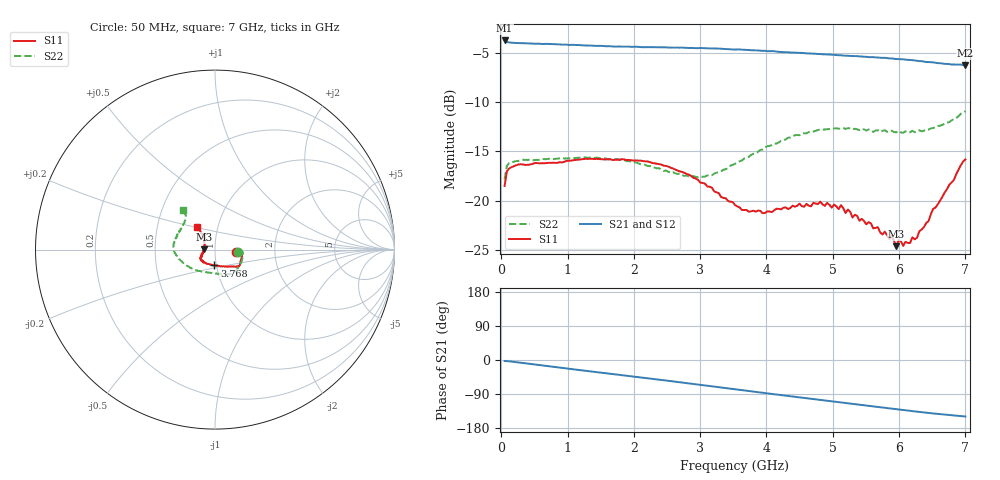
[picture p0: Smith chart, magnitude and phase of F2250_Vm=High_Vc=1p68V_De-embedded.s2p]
! Integrated Device Technology
! Corporate Headquarters
! 6024 Silver Creek Valley Road
! San Jose, CA 95138  USA
! Phone:  1-408-284-8200
! Toll Free:  1-800-223-1366
! Webpage:  http://www.idt.com/
! Timing and RF Division
! 515 Groton Road, Suite 102
! Westford, MA 01886-6024
! Device:  F2250
! Description: Voltage Variable RF Attenuator
! Frequency:  50.0 -  6000.00 MHz
! Package:  3x3 mm Thin QFN Plastic Package: 16 pin
! Ports:  2 RF, 3 DC
!  Pin  1  = GND
!  Pin  2  = NC
!  Pin  3  = RF1  = Port 1
!  Pin  4  = NC
!  Pin  5  = GND
!  Pin  6  = GND
!  Pin  7  = GND
!  Pin  8  = GND
!  Pin  9  = NC
!  Pin 10  = RF2  = Port 2
!  Pin 11  = NC
!  Pin 12  = GND
!  Pin 13  = GND
!  Pin 14  = VCNTRL
!  Pin 15  = VDD
!  Pin 16  = VMODE
! Vcntrl:  1.680 Volts
! Vmode:  +3.300 Volts
! Vdd:  +3.30  Volts
! Current:  1.326 mA
! Data:  The device was measured on a the F2250 evaluation board which has
!  individual transmission lines to the RF pins.  Data was collected
!  using a calibrated network analyzer.  The evaluation board was
!  de-embedded using a TRL calibration technique.
!  The reference plane is the edge of the package pin.
! Misc:  SN 10
!  Action Tracker AT0258
! Date Measured:  2014-11-26
! Date:  2015-10-15  MJV
! Note:
!  Integrated Device Technology supplies this data as a sample of measured
!  data at the package pin for this product.  Your particular data for this
!  product may vary.
!  Data was taken at 25 degrees C.
!  Integrated Device Technology reserves the right to change this data at anytime.
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# GHz S dB R 50
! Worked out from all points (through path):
!   201 points, 50 MHz to 7 GHz, reference 50 ohm
!   highest |S21| = -3.76 dB at 50 MHz (marker M1); lowest = -6.3 dB at 7 GHz (marker M2)
!   group delay of S21, straight-line fit = 59.8 ps
!   lowest |S11| = -24.6 dB at 5.957 GHz (marker M3), VSWR 1.12, Z = 44.5 + j0.0903 ohm
!   |S11| at or under -10 dB: start of sweep to end of sweep
!   |S22| runs from -17.9 to -10.9 dB; largest |S21 - S12| = 0.0033
!   S11 on the Smith chart (normalised r, x): 50 MHz: 1.27, -0.04; 3.768 GHz: 0.98, -0.17; 7 GHz: 0.79, +0.21
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0.05  -18.52 -6.9  -3.76 -2.5  -3.80 -2.5  -17.85 -7.2
0.08475  -17.03 -4.7  -3.92 -2.9  -3.91 -2.9  -16.47 -5.8
0.2585  -16.33 -8.2  -4.02 -6.5  -4.02 -6.5  -15.98 -11.5
1.2315  -15.80 -30.0  -4.25 -27.6  -4.28 -27.6  -15.62 -44.5
2.37825  -16.30 -38.3  -4.46 -51.8  -4.46 -51.9  -16.72 -71.5
2.969  -17.91 -47.3  -4.54 -64.8  -4.54 -64.8  -17.64 -97.9
3.525  -20.45 -73.9  -4.68 -77.2  -4.67 -77.2  -16.28 -131.2
3.76825  -21.09 -92.9  -4.75 -82.6  -4.76 -82.7  -15.37 -143.5
4.7065  -20.23 -141.1  -5.09 -103.2  -5.14 -103.1  -13.00 -175.4
5.08875  -20.87 -150.3  -5.25 -111.4  -5.25 -111.4  -12.72 175.1
5.1235  -20.47 -150.9  -5.26 -112.1  -5.28 -112.2  -12.67 174.2
5.193  -21.27 -151.5  -5.30 -113.5  -5.30 -113.6  -12.73 172.8
5.22775  -20.91 -153.5  -5.31 -114.3  -5.30 -114.4  -12.66 171.9
5.29725  -21.72 -152.9  -5.34 -115.7  -5.34 -115.8  -12.78 170.6
5.6795  -22.71 -164.1  -5.48 -123.9  -5.48 -124.0  -12.87 161.0
5.85325  -23.90 -173.7  -5.58 -127.5  -5.59 -127.6  -13.03 155.5
5.888  -23.58 -174.7  -5.58 -128.3  -5.61 -128.4  -12.91 155.7
5.9575  -24.63 179.0  -5.64 -129.7  -5.63 -129.8  -13.08 152.8
5.99225  -24.02 176.1  -5.65 -130.6  -5.65 -130.7  -12.93 152.4
6.06175  -24.60 170.8  -5.67 -131.9  -5.64 -132.0  -13.13 149.5
6.27025  -23.78 152.0  -5.82 -136.3  -5.82 -136.3  -13.03 142.9
7  -15.83 128.8  -6.26 -149.1  -6.26 -149.2  -10.93 128.6
